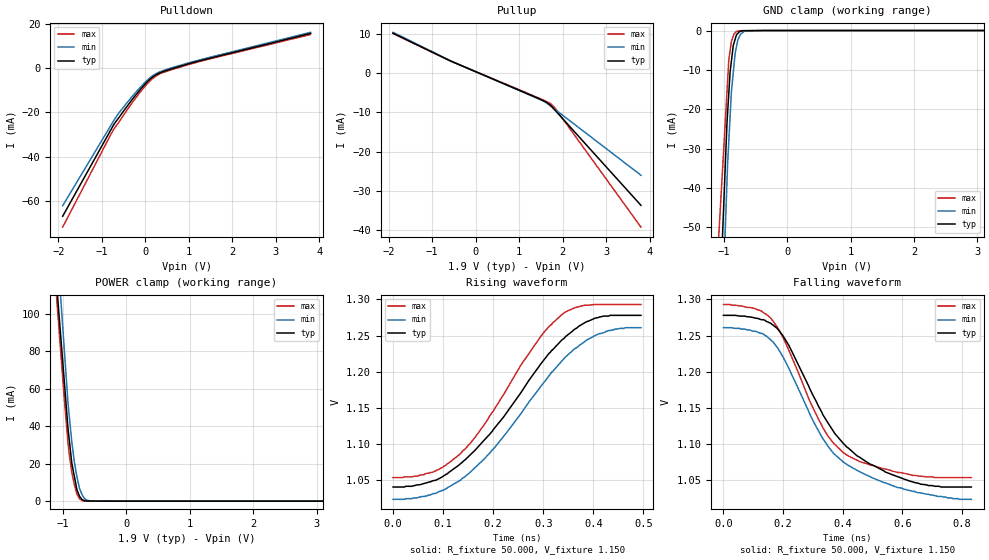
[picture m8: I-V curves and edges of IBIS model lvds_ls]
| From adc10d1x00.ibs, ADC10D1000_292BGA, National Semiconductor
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[Model]   lvds_ls
Model_type Output
Vref=1.150E+00
Rref=5.000E+01
Cref=0.000E+00
Vmeas=1.150E+00
C_comp   1.15E-12   1.15E-12   1.15E-12
[Voltage Range]   1.900E+00   1.800E+00   2.000E+00
[POWER Clamp Reference]   1.900E+00   1.800E+00   2.000E+00
[GND Clamp Reference]   0.000E+00   0.000E+00   0.000E+00
[Pullup Reference]   1.900E+00   1.800E+00   2.000E+00
[Pulldown Reference]   0.000E+00   0.000E+00   0.000E+00
[Temperature Range]   25   85   -40
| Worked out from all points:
|   slope of the pulldown table from 0 to 0.285 V, typ, clamps not added: 63.2 ohm
|   slope of the pullup table from 0 to 0.285 V, typ, clamps not added: 212 ohm
|   GND clamp passes 1 mA (typ) near -0.79 V on its own axis
|   POWER clamp passes 1 mA (typ) near -0.70 V on its own axis
|   rising waveform, R_fixture 50.000, V_fixture 1.150: 20-80 % time 160ps typ, 166ps min, 136ps max; typ from 1.04 V to 1.28 V
|   falling waveform, R_fixture 50.000, V_fixture 1.150: 20-80 % time 210ps typ, 208ps min, 166ps max; typ from 1.28 V to 1.04 V
[GND Clamp]
-2V       -453.3mA   -518.7mA   -312.7mA
-1.8V     -371.4mA   -427.3mA   -256.1mA
-950mV    -23.76mA   -38.8mA    -15.83mA
-920mV    -15.83mA   -28.04mA   -7.351mA
-900mV    -10.55mA   -21.86mA   -5.075mA
-880mV    -7.848mA   -15.67mA   -2.799mA
-850mV    -3.794mA   -10.69mA   -1.376mA
-820mV    -2.186mA   -5.717mA   -571.4uA
-800mV    -1.114mA   -4.136mA   -241.6uA
-740mV    -222.7uA   -1.029mA   -51.31uA
-640mV    -41.68uA   -74.67uA   -37.06uA
4V        0A         0A         0A
[POWER Clamp]
-2.1V     544.2mA    632.2mA    555.1mA
-1.7V     372.8mA    435.5mA    376.5mA
-1.04V    90.06mA    111mA      81.78mA
-980mV    64.35mA    81.48mA    54.99mA
-920mV    38.64mA    51.97mA    30.94mA
-900mV    32.47mA    45.16mA    24.75mA
-860mV    20.13mA    31.52mA    15.29mA
-820mV    13.13mA    20.79mA    8.74mA
-780mV    6.127mA    12.97mA    3.761mA
-700mV    862.5uA    3.573mA    318.6uA
-560mV    37.1uA     64.97uA    68.94uA
3.9V      0A         0A         0A
[Pullup]
-1.9V     10.15mA    10.38mA    10.08mA
-620mV    3.313mA    3.388mA    3.29mA
1.48V     -6.634mA   -6.717mA   -6.471mA
1.62V     -7.377mA   -7.507mA   -7.153mA
1.72V     -8.176mA   -8.34mA    -7.781mA
1.86V     -9.871mA   -9.527mA   -9.423mA
3.8V      -33.62mA   -25.97mA   -39.17mA
[Pulldown]
-1.9V     -66.97mA   -62.23mA   -71.9mA
-760mV    -26.79mA   -24.89mA   -28.85mA
-620mV    -22.73mA   -20.64mA   -24.77mA
-280mV    -13.67mA   -12.32mA   -15.07mA
-60mV     -8.443mA   -7.531mA   -9.48mA
160mV     -4.165mA   -3.577mA   -4.877mA
280mV     -2.684mA   -2.197mA   -3.187mA
400mV     -1.672mA   -1.223mA   -2.055mA
1.02V     2.066mA    2.497mA    1.726mA
3.8V      15.65mA    16.16mA    15.16mA
[Rising Waveform]
R_fixture = 50.000
V_fixture = 1.150
V_fixture_min = 1.150
V_fixture_max = 1.150
|  time   V(typ)   V(min)   V(max)
0s        1.041V     1.024V     1.054V
77ps      1.049V     1.031V     1.061V
136ps     1.074V     1.051V     1.088V
201ps     1.121V     1.094V     1.147V
295ps     1.211V     1.18V      1.249V
345ps     1.249V     1.221V     1.283V
383ps     1.268V     1.242V     1.292V
409ps     1.275V     1.252V     1.293V
442ps     1.278V     1.259V     1.293V
495ps     1.278V     1.261V     1.293V
[Falling Waveform]
R_fixture = 50.000
V_fixture = 1.150
V_fixture_min = 1.150
V_fixture_max = 1.150
|  time   V(typ)   V(min)   V(max)
0s        1.278V     1.261V     1.293V
108ps     1.274V     1.256V     1.287V
165ps     1.265V     1.242V     1.271V
220ps     1.236V     1.204V     1.229V
288ps     1.178V     1.143V     1.161V
333ps     1.141V     1.108V     1.123V
400ps     1.102V     1.076V     1.089V
494ps     1.072V     1.055V     1.071V
626ps     1.049V     1.036V     1.058V
831ps     1.041V     1.024V     1.054V
[Ramp]
dV/dt_r   1.7598E+00/1.5980E-10   1.7003E+00/1.6530E-10   1.8197E+00/1.3600E-10
dV/dt_f   1.7598E+00/2.0887E-10   1.7003E+00/2.0687E-10   1.8197E+00/1.6600E-10
R_load = 50
